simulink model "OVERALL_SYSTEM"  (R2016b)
settings: Solver=VariableStepAuto  StartTime=0.0  StopTime=12  FixedStep=0.1e-3  RelTol=1e-3
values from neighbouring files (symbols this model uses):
  beta_max = 90    [SYSTEM_PATAMETERS.m]
  beta_min = 0    [SYSTEM_PATAMETERS.m]
  beta_r = 4    [SYSTEM_PATAMETERS.m]
  c1 = 0.5    [SYSTEM_PATAMETERS.m]
  c2 = 116    [SYSTEM_PATAMETERS.m]
  c3 = 0.4    [SYSTEM_PATAMETERS.m]
  c4 = 5    [SYSTEM_PATAMETERS.m]
  c5 = 21    [SYSTEM_PATAMETERS.m]
  c6 = 0    [SYSTEM_PATAMETERS.m]
  Cdc = 0.08    [SYSTEM_PATAMETERS.m]
  Cp_max = 0.41    [SYSTEM_PATAMETERS.m]
  fn = 50    [SYSTEM_PATAMETERS.m]
  I2base = (2*Sn)/(3*V2base)    [SYSTEM_PATAMETERS.m]
  Ibase = (2*Sn)/(3*Vbase)    [SYSTEM_PATAMETERS.m]
  Idcbase = ((3/2)*Vbase*Ibase)/Vdcbase    [SYSTEM_PATAMETERS.m]
  J = Sn*2*H/(wm^2)    (= 133997.265367)    [SYSTEM_PATAMETERS.m]
  Ki = Kp/Ti    (= 750)    [SYSTEM_PATAMETERS.m]
  Ki_SSC = Kp_SSC/Ti_SSC    [SYSTEM_PATAMETERS.m]
  Kib = Kpb/Tb    (= 25)    [SYSTEM_PATAMETERS.m]
  Kibv = Kpbv/Tibv    [SYSTEM_PATAMETERS.m]
  Kidc = Kpdc/Tidc    [SYSTEM_PATAMETERS.m]
  Kiq = Kpq/Tiq    [SYSTEM_PATAMETERS.m]
  Kiw = Kpw/Tiw    (= 1)    [SYSTEM_PATAMETERS.m]
  Kp = xs_filter/(2*wbase*Ta)    (= 12.7323954474)    [SYSTEM_PATAMETERS.m]
  Kp_SSC = ls_filter/(2*wbase*Te)    [SYSTEM_PATAMETERS.m]
  Kpb = 5    [SYSTEM_PATAMETERS.m]
  Kpbv = ls_filterb/(2*wbase*Te)    [SYSTEM_PATAMETERS.m]
  Kpdc = (Vdcbase*Tc)/(V2*a*Teq)    [SYSTEM_PATAMETERS.m]
  Kpq = Tf_Q_const*rs_filter/(a*Teq)    [SYSTEM_PATAMETERS.m]
  Kpw = 4    [SYSTEM_PATAMETERS.m]
  lambda_opt = 7.95    [SYSTEM_PATAMETERS.m]
  ls = Ls/Lbase    [SYSTEM_PATAMETERS.m]
  ls_filter = Ls_filter/Lbase    [SYSTEM_PATAMETERS.m]
  Ls_filter = Xs_filter/we    [SYSTEM_PATAMETERS.m]
  polepairs = poles/2    (= 115)    [SYSTEM_PATAMETERS.m]
  psim_pu = psim/psibase    [SYSTEM_PATAMETERS.m]
  r = 26    [SYSTEM_PATAMETERS.m]
  rho = 1.225    [SYSTEM_PATAMETERS.m]
  Rs = rs*Zbase    [SYSTEM_PATAMETERS.m]
  Rs_filter = rs_filter*Zbase    [SYSTEM_PATAMETERS.m]
  Sn = 250e3    (= 250000)    [SYSTEM_PATAMETERS.m]
  Ta = Tsw/2    (= 0.0001)    [SYSTEM_PATAMETERS.m]
  Ts = 1e-5    (= 1e-05)    [SYSTEM_PATAMETERS.m]
  V2 = 400    [SYSTEM_PATAMETERS.m]
  V2base = V2*sqrt(2)/sqrt(3)    [SYSTEM_PATAMETERS.m]
  Vbase = V1*sqrt(2)/sqrt(3)    [SYSTEM_PATAMETERS.m]
  Vdcbase = 3*Vbase    [SYSTEM_PATAMETERS.m]
  w2base = 2*pi*fn    (= 314.159265359)    [SYSTEM_PATAMETERS.m]
  wbase = 2*pi*fn    (= 314.159265359)    [SYSTEM_PATAMETERS.m]
  wm = nm*pi/30    (= 2.73181969877)    [SYSTEM_PATAMETERS.m]
undefined symbols (not defined in the file or in its folder): bridge, by, dend, DiscIntNeverNeededParam, established, Flux, h, Ion, K, Ld, linkage, Lithium, Lq, magnets, numd, phase, Pm0, pulses, sigbuilder_block, Td, Three, Tlim, Tr, V
libraries: powerlib x32, powerlib_meascontrol x14, simulink x10, powerlib_extras x2, sps_avr x1, electricdrivelib x1
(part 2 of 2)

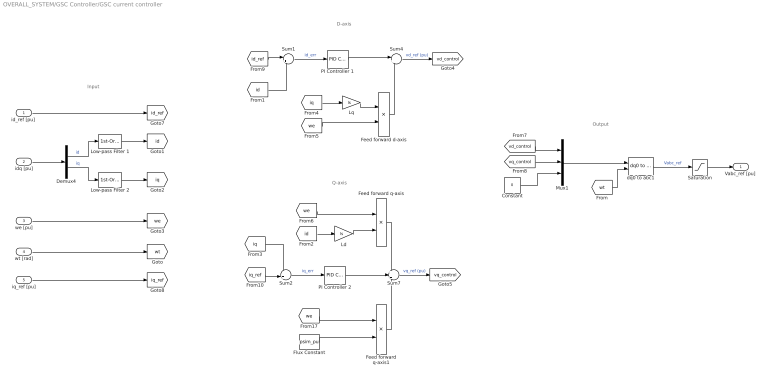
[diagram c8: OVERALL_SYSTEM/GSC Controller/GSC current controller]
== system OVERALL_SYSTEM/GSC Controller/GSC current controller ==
  note: D-axis
  note: Q-axis
  note: Input
  note: Output
  "id_ref [pu] " : Inport
  idq [pu] : Inport  Port=2
  we [pu] : Inport  Port=3
  wt [rad] : Inport  Port=4
  iq_ref [pu] : Inport  Port=5
  Constant : Constant  Value=0
  Demux4 : Demux  Outputs=2
  Feed forward d-axis : Product
  Feed forward q-axis : Product
  Feed forward q-axis1 : Product
  Flux Constant : Constant  Value=psim_pu
  Ld : Gain  Gain=ls
  Low-pass Filter 1 : powerlib_extras/Control  Blocks/1st-Order  Filter  FilterType=Lowpass  Tc=3e-4  Initialize=off  Vac_Init=[0.8 -25 50]  Vdc_Init=0  PlotResponse=off  param1=[1 2000 1]
  Low-pass Filter 2 : powerlib_extras/Control  Blocks/1st-Order  Filter  FilterType=Lowpass  Tc=3e-4  Initialize=off  Vac_Init=[0.8 -25 50]  Vdc_Init=0  PlotResponse=off  param1=[1 2000 1]
  Lq : Gain  Gain=ls
  Mux1 : Mux  Inputs=3
  PI Controller 1 : simulink/Continuous/PID Controller  Controller=PI  TimeDomain=Continuous-time  SampleTime=-1  IntegratorMethod=Forward Euler  FilterMethod=Forward Euler  Form=Parallel  UseFilter=on  ControllerParametersSource=internal  P=Kp  I=Ki  D=0  N=100  InitialConditionSource=internal  InitialConditionForIntegrator=0  InitialConditionForFilter=0  ExternalReset=none  LimitOutput=off  UpperSaturationLimit=inf  LowerSaturationLimit=-inf  LinearizeAsGain=on  AntiWindupMode=none  Kb=1  TrackingMode=off  Kt=1  PParamMin=[]  PParamMax=[]  IParamMin=[]  IParamMax=[]  DParamMin=[]  DParamMax=[]  NParamMin=[]  NParamMax=[]  KbParamMin=[]  KbParamMax=[]  KtParamMin=[]  KtParamMax=[]  POutMin=[]  POutMax=[]  IOutMin=[]  IOutMax=[]  DOutMin=[]  DOutMax=[]  NOutMin=[]  NOutMax=[]  KbOutMin=[]  KbOutMax=[]  KtOutMin=[]  KtOutMax=[]  IntegratorOutMin=[]  IntegratorOutMax=[]  FilterOutMin=[]  FilterOutMax=[]  SumOutMin=[]  SumOutMax=[]  SumI1OutMin=[]  SumI1OutMax=[]  SumI2OutMin=[]  SumI2OutMax=[]  SumI3OutMin=[]  SumI3OutMax=[]  SumDOutMin=[]  SumDOutMax=[]  SaturationOutMin=[]  SaturationOutMax=[]  IntegratorContinuousStateAttributes=''  IntegratorStateMustResolveToSignalObject=off  IntegratorRTWStateStorageClass=Auto  FilterContinuousStateAttributes=''  FilterStateMustResolveToSignalObject=off  FilterRTWStateStorageClass=Auto  DifferentiatorICPrevScaledInput=0  DifferentiatorOutMin=[]  DifferentiatorOutMax=[]
  PI Controller 2 : simulink/Continuous/PID Controller  Controller=PI  TimeDomain=Continuous-time  SampleTime=-1  IntegratorMethod=Forward Euler  FilterMethod=Forward Euler  Form=Parallel  UseFilter=on  ControllerParametersSource=internal  P=Kp  I=Ki  D=0  N=100  InitialConditionSource=internal  InitialConditionForIntegrator=0  InitialConditionForFilter=0  ExternalReset=none  LimitOutput=off  UpperSaturationLimit=inf  LowerSaturationLimit=-inf  LinearizeAsGain=on  AntiWindupMode=none  Kb=1  TrackingMode=off  Kt=1  PParamMin=[]  PParamMax=[]  IParamMin=[]  IParamMax=[]  DParamMin=[]  DParamMax=[]  NParamMin=[]  NParamMax=[]  KbParamMin=[]  KbParamMax=[]  KtParamMin=[]  KtParamMax=[]  POutMin=[]  POutMax=[]  IOutMin=[]  IOutMax=[]  DOutMin=[]  DOutMax=[]  NOutMin=[]  NOutMax=[]  KbOutMin=[]  KbOutMax=[]  KtOutMin=[]  KtOutMax=[]  IntegratorOutMin=[]  IntegratorOutMax=[]  FilterOutMin=[]  FilterOutMax=[]  SumOutMin=[]  SumOutMax=[]  SumI1OutMin=[]  SumI1OutMax=[]  SumI2OutMin=[]  SumI2OutMax=[]  SumI3OutMin=[]  SumI3OutMax=[]  SumDOutMin=[]  SumDOutMax=[]  SaturationOutMin=[]  SaturationOutMax=[]  IntegratorContinuousStateAttributes=''  IntegratorStateMustResolveToSignalObject=off  IntegratorRTWStateStorageClass=Auto  FilterContinuousStateAttributes=''  FilterStateMustResolveToSignalObject=off  FilterRTWStateStorageClass=Auto  DifferentiatorICPrevScaledInput=0  DifferentiatorOutMin=[]  DifferentiatorOutMax=[]
  Saturation : Saturate  UpperLimit=1  LowerLimit=-1
  Sum1 : Sum  Inputs=|+-
  Sum2 : Sum  Inputs=-+|
  Sum4 : Sum  Inputs=|+-
  Sum7 : Sum  Inputs=+++
  dq0 to abc1 : powerlib_meascontrol/Transformations/dq0 to abc  Alignment=Aligned with phase A axis
  "Vabc_ref [pu] " : Outport
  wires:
  PI Controller 2/1 -> Sum7/2
  Demux4/1 -> Low-pass Filter 1/1  "id"
  "id_ref [pu] "/1 -> [id_ref]
  Constant/1 -> Mux1/3
  Sum2/1 -> PI Controller 2/1  "iq_err"
  dq0 to abc1/1 -> Saturation/1  "Vabc_ref"
  Sum4/1 -> [vd_control]  "vd_ref (pu)"
  Feed forward q-axis/1 -> Sum7/1
  Mux1/1 -> dq0 to abc1/1
  Sum7/1 -> [vq_control]  "vq_ref (pu)"
  Ld/1 -> Feed forward q-axis/2
  Sum1/1 -> PI Controller 1/1  "id_err"
  Lq/1 -> Feed forward d-axis/1
  PI Controller 1/1 -> Sum4/1
  Feed forward d-axis/1 -> Sum4/2
  idq [pu]/1 -> Demux4/1
  wt [rad]/1 -> [wt]
  [wt] -> dq0 to abc1/2
  Demux4/2 -> Low-pass Filter 2/1  "iq"
  [id] -> Ld/1
  [iq] -> Lq/1
  we [pu]/1 -> [we]
  [we] -> Feed forward d-axis/2
  [we] -> Feed forward q-axis/1
  [vd_control] -> Mux1/1
  [vq_control] -> Mux1/2
  Saturation/1 -> "Vabc_ref [pu] "/1
  Flux Constant/1 -> Feed forward q-axis1/2
  [we] -> Feed forward q-axis1/1
  Feed forward q-axis1/1 -> Sum7/3
  [iq] -> Sum2/1
  [id] -> Sum1/2
  iq_ref [pu]/1 -> [iq_ref]
  Low-pass Filter 1/1 -> [id]
  Low-pass Filter 2/1 -> [iq]
  [id_ref] -> Sum1/1
  [iq_ref] -> Sum2/2

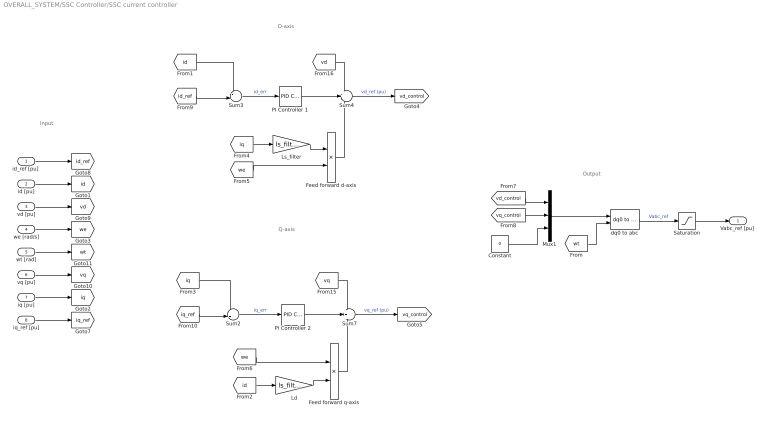
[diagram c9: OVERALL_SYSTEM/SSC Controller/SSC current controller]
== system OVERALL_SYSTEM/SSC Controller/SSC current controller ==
  note: D-axis
  note: Q-axis
  note: Input
  note: Output
  "id_ref [pu] " : Inport
  id [pu] : Inport  Port=2
  vd [pu] : Inport  Port=3
  we [rad/s] : Inport  Port=4
  wt [rad] : Inport  Port=5
  vq [pu] : Inport  Port=6
  iq [pu] : Inport  Port=7
  iq_ref [pu] : Inport  Port=8
  Constant : Constant  Value=0
  Feed forward d-axis : Product
  Feed forward q-axis : Product
  Ld : Gain  Gain=ls_filter
  Ls_filter : Gain  Gain=ls_filter
  Mux1 : Mux  Inputs=3
  PI Controller 1 : simulink/Continuous/PID Controller  Controller=PI  TimeDomain=Continuous-time  SampleTime=-1  IntegratorMethod=Forward Euler  FilterMethod=Forward Euler  Form=Parallel  UseFilter=on  ControllerParametersSource=internal  P=Kp_SSC  I=Ki_SSC  D=0.05  N=1  InitialConditionSource=internal  InitialConditionForIntegrator=0  InitialConditionForFilter=0  ExternalReset=none  LimitOutput=off  UpperSaturationLimit=inf  LowerSaturationLimit=-inf  LinearizeAsGain=on  AntiWindupMode=none  Kb=1  TrackingMode=off  Kt=1  PParamMin=[]  PParamMax=[]  IParamMin=[]  IParamMax=[]  DParamMin=[]  DParamMax=[]  NParamMin=[]  NParamMax=[]  KbParamMin=[]  KbParamMax=[]  KtParamMin=[]  KtParamMax=[]  POutMin=[]  POutMax=[]  IOutMin=[]  IOutMax=[]  DOutMin=[]  DOutMax=[]  NOutMin=[]  NOutMax=[]  KbOutMin=[]  KbOutMax=[]  KtOutMin=[]  KtOutMax=[]  IntegratorOutMin=[]  IntegratorOutMax=[]  FilterOutMin=[]  FilterOutMax=[]  SumOutMin=[]  SumOutMax=[]  SumI1OutMin=[]  SumI1OutMax=[]  SumI2OutMin=[]  SumI2OutMax=[]  SumI3OutMin=[]  SumI3OutMax=[]  SumDOutMin=[]  SumDOutMax=[]  SaturationOutMin=[]  SaturationOutMax=[]  IntegratorContinuousStateAttributes=''  IntegratorStateMustResolveToSignalObject=off  IntegratorRTWStateStorageClass=Auto  FilterContinuousStateAttributes=''  FilterStateMustResolveToSignalObject=off  FilterRTWStateStorageClass=Auto  DifferentiatorICPrevScaledInput=0  DifferentiatorOutMin=[]  DifferentiatorOutMax=[]
  PI Controller 2 : simulink/Continuous/PID Controller  Controller=PI  TimeDomain=Continuous-time  SampleTime=-1  IntegratorMethod=Forward Euler  FilterMethod=Forward Euler  Form=Parallel  UseFilter=on  ControllerParametersSource=internal  P=Kp_SSC  I=Ki_SSC  D=0  N=100  InitialConditionSource=internal  InitialConditionForIntegrator=0  InitialConditionForFilter=0  ExternalReset=none  LimitOutput=off  UpperSaturationLimit=inf  LowerSaturationLimit=-inf  LinearizeAsGain=on  AntiWindupMode=none  Kb=1  TrackingMode=off  Kt=1  PParamMin=[]  PParamMax=[]  IParamMin=[]  IParamMax=[]  DParamMin=[]  DParamMax=[]  NParamMin=[]  NParamMax=[]  KbParamMin=[]  KbParamMax=[]  KtParamMin=[]  KtParamMax=[]  POutMin=[]  POutMax=[]  IOutMin=[]  IOutMax=[]  DOutMin=[]  DOutMax=[]  NOutMin=[]  NOutMax=[]  KbOutMin=[]  KbOutMax=[]  KtOutMin=[]  KtOutMax=[]  IntegratorOutMin=[]  IntegratorOutMax=[]  FilterOutMin=[]  FilterOutMax=[]  SumOutMin=[]  SumOutMax=[]  SumI1OutMin=[]  SumI1OutMax=[]  SumI2OutMin=[]  SumI2OutMax=[]  SumI3OutMin=[]  SumI3OutMax=[]  SumDOutMin=[]  SumDOutMax=[]  SaturationOutMin=[]  SaturationOutMax=[]  IntegratorContinuousStateAttributes=''  IntegratorStateMustResolveToSignalObject=off  IntegratorRTWStateStorageClass=Auto  FilterContinuousStateAttributes=''  FilterStateMustResolveToSignalObject=off  FilterRTWStateStorageClass=Auto  DifferentiatorICPrevScaledInput=0  DifferentiatorOutMin=[]  DifferentiatorOutMax=[]
  Saturation : Saturate  UpperLimit=1  LowerLimit=-1
  Sum2 : Sum  Inputs=-+|
  Sum3 : Sum  Inputs=-+|
  Sum4 : Sum  Inputs=++-
  Sum7 : Sum  Inputs=+++
  dq0 to abc : powerlib_meascontrol/Transformations/dq0 to abc  Alignment=90 degrees behind phase A axis
  "Vabc_ref [pu] " : Outport
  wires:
  PI Controller 2/1 -> Sum7/2
  "id_ref [pu] "/1 -> [id_ref]
  Constant/1 -> Mux1/3
  Sum2/1 -> PI Controller 2/1  "iq_err"
  dq0 to abc/1 -> Saturation/1  "Vabc_ref"
  Sum4/1 -> [vd_control]  "vd_ref (pu)"
  Mux1/1 -> dq0 to abc/1
  Sum7/1 -> [vq_control]  "vq_ref (pu)"
  Sum3/1 -> PI Controller 1/1  "id_err"
  iq_ref [pu]/1 -> [iq_ref]
  Ls_filter/1 -> Feed forward d-axis/1
  [wt] -> dq0 to abc/2
  [iq] -> Sum2/1
  [iq] -> Ls_filter/1
  [we] -> Feed forward d-axis/2
  [vd_control] -> Mux1/1
  [vq_control] -> Mux1/2
  Saturation/1 -> "Vabc_ref [pu] "/1
  Feed forward d-axis/1 -> Sum4/3
  PI Controller 1/1 -> Sum4/2
  [vd] -> Sum4/1
  id [pu]/1 -> [id]
  iq [pu]/1 -> [iq]
  wt [rad]/1 -> [wt]
  vd [pu]/1 -> [vd]
  vq [pu]/1 -> [vq]
  we [rad/s]/1 -> [we]
  [id] -> Sum3/1
  [vq] -> Sum7/1
  [id_ref] -> Sum3/2
  [iq_ref] -> Sum2/2
  Feed forward q-axis/1 -> Sum7/3
  Ld/1 -> Feed forward q-axis/2
  [id] -> Ld/1
  [we] -> Feed forward q-axis/1

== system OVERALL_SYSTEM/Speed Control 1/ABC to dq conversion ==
  Iabc : Inport
  Teta : Inport  Port=2
  Fcn : Fcn  Expr=sin(u)
  Fcn1 : Fcn  Expr=cos(u)
  Gain : Gain  Gain=2/3
  Gain1 : Gain  Gain=2/3
  Mux : Mux  Inputs=[1 1 3]
  id : Fcn  Expr=u[1]*u[3]+(1.7320508*u[2]-u[1])*u[4]*0.5+(-u[1]-1.7320508*u[2])*u[5]*0.5
  iq : Fcn  Expr=-u[2]*u[3]+(u[2]+1.7320508*u[1])*u[4]*0.5+(u[2]-1.7320508*u[1])*u[5]*0.5
  Id : Outport  InitialOutput=0
  Iq : Outport  Port=2  InitialOutput=0
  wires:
  Fcn/1 -> Mux/2
  Fcn1/1 -> Mux/1
  Teta/1 -> Fcn1/1, Fcn/1
  Mux/1 -> iq/1, id/1
  Iabc/1 -> Mux/3
  iq/1 -> Gain1/1
  id/1 -> Gain/1
  Gain/1 -> Id/1
  Gain1/1 -> Iq/1

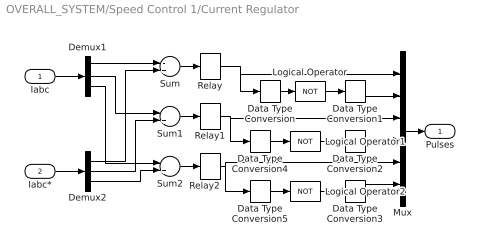
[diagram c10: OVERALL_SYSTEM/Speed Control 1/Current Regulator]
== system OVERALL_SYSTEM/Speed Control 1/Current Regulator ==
  Iabc : Inport
  Iabc* : Inport  Port=2
  Data Type Conversion : DataTypeConversion  OutDataTypeStr=boolean
  Data Type Conversion1 : DataTypeConversion  OutDataTypeStr=double
  Data Type Conversion2 : DataTypeConversion  OutDataTypeStr=double
  Data Type Conversion3 : DataTypeConversion  OutDataTypeStr=double
  Data Type Conversion4 : DataTypeConversion  OutDataTypeStr=boolean
  Data Type Conversion5 : DataTypeConversion  OutDataTypeStr=boolean
  Demux1 : Demux  Outputs=3
  Demux2 : Demux  Outputs=3
  Logical Operator : Logic  Operator=NOT
  Logical Operator1 : Logic  Operator=NOT
  Logical Operator2 : Logic  Operator=NOT
  Mux : Mux  Inputs=6
  Relay : Relay  OnSwitchValue=h/2  OffSwitchValue=-h/2
  Relay1 : Relay  OnSwitchValue=h/2  OffSwitchValue=-h/2
  Relay2 : Relay  OnSwitchValue=h/2  OffSwitchValue=-h/2
  Sum : Sum  Inputs=-+
  Sum1 : Sum  Inputs=-+
  Sum2 : Sum  Inputs=-+
  Pulses : Outport  InitialOutput=0
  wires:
  Sum/1 -> Relay/1
  Sum1/1 -> Relay1/1
  Demux1/1 -> Sum/1
  Demux1/2 -> Sum1/1
  Mux/1 -> Pulses/1
  Iabc/1 -> Demux1/1
  Sum2/1 -> Relay2/1
  Demux1/3 -> Sum2/1
  Demux2/3 -> Sum2/2
  Demux2/2 -> Sum1/2
  Demux2/1 -> Sum/2
  Iabc*/1 -> Demux2/1
  Relay/1 -> Mux/1, Data Type Conversion/1
  Relay1/1 -> Mux/3, Data Type Conversion4/1
  Relay2/1 -> Mux/5, Data Type Conversion5/1
  Data Type Conversion/1 -> Logical Operator/1
  Logical Operator/1 -> Data Type Conversion1/1
  Data Type Conversion1/1 -> Mux/2
  Logical Operator1/1 -> Data Type Conversion2/1
  Data Type Conversion2/1 -> Mux/4
  Logical Operator2/1 -> Data Type Conversion3/1
  Data Type Conversion3/1 -> Mux/6
  Data Type Conversion4/1 -> Logical Operator1/1
  Data Type Conversion5/1 -> Logical Operator2/1

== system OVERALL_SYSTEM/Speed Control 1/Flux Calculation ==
  note: Phir = Lm *Id / (1 +Tr .s)
  note: Lm = 34.7 mH
  note: Lr = Ll'r +Lm = 0.8 +34.7= 35.5 mH
  note: Tr = Lr / Rr = 0.1557 s
  note: Rr = 0.228 ohms
  Id : Inport
  Discrete Tranfer Function : Subsystem
  Lm : Gain  Gain=34.7e-3
  Phir : Outport
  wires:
  Discrete Tranfer Function/1(Out) -> Phir/1
  Id/1 -> Lm/1
  Lm/1 -> Discrete Tranfer Function/1(In)

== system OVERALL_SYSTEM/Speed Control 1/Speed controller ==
  w : Inport
  w* : Inport  Port=2
  Discrete-Time Integrator : DiscreteIntegrator  IntegratorMethod=Integration: Trapezoidal  SampleTime=Ts  LimitOutput=on  UpperSaturationLimit=Tlim  LowerSaturationLimit=-Tlim  ICPrevOutput=DiscIntNeverNeededParam  ICPrevScaledInput=DiscIntNeverNeededParam
  Gain : Gain  Gain=Ki
  Gain1 : Gain  Gain=Kp
  Saturation : Saturate  UpperLimit=Tlim  LowerLimit=-Tlim
  Sum1 : Sum  Inputs=+-
  Sum2 : Sum
  Te* : Outport  InitialOutput=0
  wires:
  Gain1/1 -> Sum2/1
  Gain/1 -> Discrete-Time Integrator/1
  Sum1/1 -> Gain/1, Gain1/1
  Discrete-Time Integrator/1 -> Sum2/2
  Sum2/1 -> Saturation/1
  Saturation/1 -> Te*/1
  w/1 -> Sum1/2
  w*/1 -> Sum1/1

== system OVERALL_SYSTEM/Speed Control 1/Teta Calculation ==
  note: Teta= Electrical angle= integ ( wr + wm)
  note: wr = Rotor frequency (rad/s) = Lm *Iq / ( Tr * Phir)
  note: Lm = 34.7 mH
  note: Rr= 0.228 ohms
  note: Lr = Ll'r +Lm = 0.8 +34.7= 35.5 mH
  note: wm= Rotor mechanical speed (rad/s)
  note: Tr = Lr / Rr = 0.1557 s
  Phir : Inport
  wm : Inport  Port=2
  Iq : Inport  Port=3
  Discrete-Time Integrator : DiscreteIntegrator  SampleTime=Ts  ICPrevOutput=DiscIntNeverNeededParam  ICPrevScaledInput=DiscIntNeverNeededParam
  Fcn : Fcn  Expr=34.7e-3*u[1]/(u[2]*0.1557+1e-3)
  Gain2 : Gain
  Gain3 : Gain  Gain=2
  Mux : Mux  Inputs=2
  Sum : Sum
  Teta : Outport  InitialOutput=0
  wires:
  Discrete-Time Integrator/1 -> Teta/1
  Sum/1 -> Discrete-Time Integrator/1
  Gain3/1 -> Sum/2
  Gain2/1 -> Sum/1
  wm/1 -> Gain3/1
  Fcn/1 -> Gain2/1
  Phir/1 -> Mux/2
  Iq/1 -> Mux/1
  Mux/1 -> Fcn/1

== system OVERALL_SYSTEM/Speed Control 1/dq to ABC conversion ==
  Teta : Inport
  Id* : Inport  Port=2
  Iq* : Inport  Port=3
  Fcn : Fcn  Expr=sin(u)
  Fcn1 : Fcn  Expr=cos(u)
  Gain2 : Gain
  Gain3 : Gain
  Gain4 : Gain
  Mux : Mux
  Mux2 : Mux  Inputs=3
  ia : Fcn  Expr=-u[3]*u[2] + u[4]*u[1]
  ib : Fcn  Expr=(-u[1]+1.7320508*u[2])*u[4]*0.5+(u[2]+1.7320508*u[1])*u[3]*0.5
  ic : Sum  Inputs=--
  Iabc* : Outport  InitialOutput=0
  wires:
  Fcn/1 -> Mux/2
  Fcn1/1 -> Mux/1
  Mux2/1 -> Iabc*/1
  Mux/1 -> ib/1, ia/1
  Teta/1 -> Fcn1/1, Fcn/1
  Iq*/1 -> Mux/3
  Id*/1 -> Mux/4
  Gain3/1 -> Mux2/2
  ic/1 -> Gain4/1
  Gain4/1 -> Mux2/3
  Gain2/1 -> Mux2/1
  ia/1 -> Gain2/1, ic/2
  ib/1 -> Gain3/1, ic/1

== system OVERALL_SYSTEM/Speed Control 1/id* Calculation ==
  note: Id* = Phir*/ Lm
  note: Lm= 34.7 mH
  Phir* : Inport
  KF : Gain  Gain=1/34.7e-3
  Id* : Outport
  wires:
  KF/1 -> Id*/1
  Phir*/1 -> KF/1

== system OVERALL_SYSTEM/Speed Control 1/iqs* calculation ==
  note: Iq= ( 2/3) * (2/p) * ( Lr/Lm) * (Te / Phir)
  note: Lm = 34.7 mH
  note: Lr = Ll'r +Lm = 0.8 +34.7= 35.5 mH
  note: p= nb of poles = 4
  note: Iq= 0.341 * (Te / Phir)
  Phir : Inport
  Te* : Inport  Port=2
  Fcn : Fcn  Expr=u[1]*0.341/(u[2]+1e-3)
  Mux1 : Mux  Inputs=2
  Iq* : Outport  InitialOutput=0
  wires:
  Phir/1 -> Mux1/2
  Fcn/1 -> Iq*/1
  Te*/1 -> Mux1/1
  Mux1/1 -> Fcn/1

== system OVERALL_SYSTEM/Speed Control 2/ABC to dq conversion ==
  Iabc : Inport
  Teta : Inport  Port=2
  Fcn : Fcn  Expr=sin(u)
  Fcn1 : Fcn  Expr=cos(u)
  Gain : Gain  Gain=2/3
  Gain1 : Gain  Gain=2/3
  Mux : Mux  Inputs=[1 1 3]
  id : Fcn  Expr=u[1]*u[3]+(1.7320508*u[2]-u[1])*u[4]*0.5+(-u[1]-1.7320508*u[2])*u[5]*0.5
  iq : Fcn  Expr=-u[2]*u[3]+(u[2]+1.7320508*u[1])*u[4]*0.5+(u[2]-1.7320508*u[1])*u[5]*0.5
  Id : Outport  InitialOutput=0
  Iq : Outport  Port=2  InitialOutput=0
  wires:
  Fcn/1 -> Mux/2
  Fcn1/1 -> Mux/1
  Teta/1 -> Fcn1/1, Fcn/1
  Mux/1 -> iq/1, id/1
  Iabc/1 -> Mux/3
  iq/1 -> Gain1/1
  id/1 -> Gain/1
  Gain/1 -> Id/1
  Gain1/1 -> Iq/1

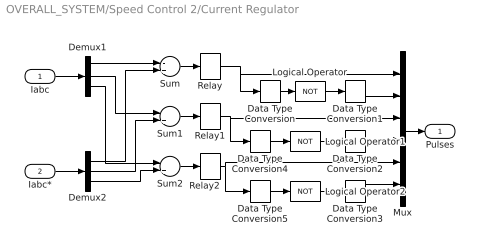
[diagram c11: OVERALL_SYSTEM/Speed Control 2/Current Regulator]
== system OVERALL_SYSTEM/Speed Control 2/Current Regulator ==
  Iabc : Inport
  Iabc* : Inport  Port=2
  Data Type Conversion : DataTypeConversion  OutDataTypeStr=boolean
  Data Type Conversion1 : DataTypeConversion  OutDataTypeStr=double
  Data Type Conversion2 : DataTypeConversion  OutDataTypeStr=double
  Data Type Conversion3 : DataTypeConversion  OutDataTypeStr=double
  Data Type Conversion4 : DataTypeConversion  OutDataTypeStr=boolean
  Data Type Conversion5 : DataTypeConversion  OutDataTypeStr=boolean
  Demux1 : Demux  Outputs=3
  Demux2 : Demux  Outputs=3
  Logical Operator : Logic  Operator=NOT
  Logical Operator1 : Logic  Operator=NOT
  Logical Operator2 : Logic  Operator=NOT
  Mux : Mux  Inputs=6
  Relay : Relay  OnSwitchValue=h/2  OffSwitchValue=-h/2
  Relay1 : Relay  OnSwitchValue=h/2  OffSwitchValue=-h/2
  Relay2 : Relay  OnSwitchValue=h/2  OffSwitchValue=-h/2
  Sum : Sum  Inputs=-+
  Sum1 : Sum  Inputs=-+
  Sum2 : Sum  Inputs=-+
  Pulses : Outport  InitialOutput=0
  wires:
  Sum/1 -> Relay/1
  Sum1/1 -> Relay1/1
  Demux1/1 -> Sum/1
  Demux1/2 -> Sum1/1
  Mux/1 -> Pulses/1
  Iabc/1 -> Demux1/1
  Sum2/1 -> Relay2/1
  Demux1/3 -> Sum2/1
  Demux2/3 -> Sum2/2
  Demux2/2 -> Sum1/2
  Demux2/1 -> Sum/2
  Iabc*/1 -> Demux2/1
  Relay/1 -> Mux/1, Data Type Conversion/1
  Relay1/1 -> Mux/3, Data Type Conversion4/1
  Relay2/1 -> Mux/5, Data Type Conversion5/1
  Data Type Conversion/1 -> Logical Operator/1
  Logical Operator/1 -> Data Type Conversion1/1
  Data Type Conversion1/1 -> Mux/2
  Logical Operator1/1 -> Data Type Conversion2/1
  Data Type Conversion2/1 -> Mux/4
  Logical Operator2/1 -> Data Type Conversion3/1
  Data Type Conversion3/1 -> Mux/6
  Data Type Conversion4/1 -> Logical Operator1/1
  Data Type Conversion5/1 -> Logical Operator2/1

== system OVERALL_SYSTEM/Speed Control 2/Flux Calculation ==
  note: Phir = Lm *Id / (1 +Tr .s)
  note: Lm = 34.7 mH
  note: Lr = Ll'r +Lm = 0.8 +34.7= 35.5 mH
  note: Tr = Lr / Rr = 0.1557 s
  note: Rr = 0.228 ohms
  Id : Inport
  Discrete Tranfer Function : Subsystem
  Lm : Gain  Gain=34.7e-3
  Phir : Outport
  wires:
  Discrete Tranfer Function/1(Out) -> Phir/1
  Id/1 -> Lm/1
  Lm/1 -> Discrete Tranfer Function/1(In)

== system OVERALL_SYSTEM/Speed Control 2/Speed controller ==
  w : Inport
  w* : Inport  Port=2
  Discrete-Time Integrator : DiscreteIntegrator  IntegratorMethod=Integration: Trapezoidal  SampleTime=Ts  LimitOutput=on  UpperSaturationLimit=Tlim  LowerSaturationLimit=-Tlim  ICPrevOutput=DiscIntNeverNeededParam  ICPrevScaledInput=DiscIntNeverNeededParam
  Gain : Gain  Gain=Ki
  Gain1 : Gain  Gain=Kp
  Saturation : Saturate  UpperLimit=Tlim  LowerLimit=-Tlim
  Sum1 : Sum  Inputs=+-
  Sum2 : Sum
  Te* : Outport  InitialOutput=0
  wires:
  Gain1/1 -> Sum2/1
  Gain/1 -> Discrete-Time Integrator/1
  Sum1/1 -> Gain/1, Gain1/1
  Discrete-Time Integrator/1 -> Sum2/2
  Sum2/1 -> Saturation/1
  Saturation/1 -> Te*/1
  w/1 -> Sum1/2
  w*/1 -> Sum1/1

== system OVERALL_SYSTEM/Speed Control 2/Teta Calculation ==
  note: Teta= Electrical angle= integ ( wr + wm)
  note: wr = Rotor frequency (rad/s) = Lm *Iq / ( Tr * Phir)
  note: Lm = 34.7 mH
  note: Rr= 0.228 ohms
  note: Lr = Ll'r +Lm = 0.8 +34.7= 35.5 mH
  note: wm= Rotor mechanical speed (rad/s)
  note: Tr = Lr / Rr = 0.1557 s
  Phir : Inport
  wm : Inport  Port=2
  Iq : Inport  Port=3
  Discrete-Time Integrator : DiscreteIntegrator  SampleTime=Ts  ICPrevOutput=DiscIntNeverNeededParam  ICPrevScaledInput=DiscIntNeverNeededParam
  Fcn : Fcn  Expr=34.7e-3*u[1]/(u[2]*0.1557+1e-3)
  Gain2 : Gain
  Gain3 : Gain  Gain=2
  Mux : Mux  Inputs=2
  Sum : Sum
  Teta : Outport  InitialOutput=0
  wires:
  Discrete-Time Integrator/1 -> Teta/1
  Sum/1 -> Discrete-Time Integrator/1
  Gain3/1 -> Sum/2
  Gain2/1 -> Sum/1
  wm/1 -> Gain3/1
  Fcn/1 -> Gain2/1
  Phir/1 -> Mux/2
  Iq/1 -> Mux/1
  Mux/1 -> Fcn/1

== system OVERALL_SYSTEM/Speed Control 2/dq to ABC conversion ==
  Teta : Inport
  Id* : Inport  Port=2
  Iq* : Inport  Port=3
  Fcn : Fcn  Expr=sin(u)
  Fcn1 : Fcn  Expr=cos(u)
  Gain2 : Gain
  Gain3 : Gain
  Gain4 : Gain
  Mux : Mux
  Mux2 : Mux  Inputs=3
  ia : Fcn  Expr=-u[3]*u[2] + u[4]*u[1]
  ib : Fcn  Expr=(-u[1]+1.7320508*u[2])*u[4]*0.5+(u[2]+1.7320508*u[1])*u[3]*0.5
  ic : Sum  Inputs=--
  Iabc* : Outport  InitialOutput=0
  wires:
  Fcn/1 -> Mux/2
  Fcn1/1 -> Mux/1
  Mux2/1 -> Iabc*/1
  Mux/1 -> ib/1, ia/1
  Teta/1 -> Fcn1/1, Fcn/1
  Iq*/1 -> Mux/3
  Id*/1 -> Mux/4
  Gain3/1 -> Mux2/2
  ic/1 -> Gain4/1
  Gain4/1 -> Mux2/3
  Gain2/1 -> Mux2/1
  ia/1 -> Gain2/1, ic/2
  ib/1 -> Gain3/1, ic/1

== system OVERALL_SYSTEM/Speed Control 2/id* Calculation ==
  note: Id* = Phir*/ Lm
  note: Lm= 34.7 mH
  Phir* : Inport
  KF : Gain  Gain=1/34.7e-3
  Id* : Outport
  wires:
  KF/1 -> Id*/1
  Phir*/1 -> KF/1

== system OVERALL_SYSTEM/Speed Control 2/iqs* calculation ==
  note: Iq= ( 2/3) * (2/p) * ( Lr/Lm) * (Te / Phir)
  note: Lm = 34.7 mH
  note: Lr = Ll'r +Lm = 0.8 +34.7= 35.5 mH
  note: p= nb of poles = 4
  note: Iq= 0.341 * (Te / Phir)
  Phir : Inport
  Te* : Inport  Port=2
  Fcn : Fcn  Expr=u[1]*0.341/(u[2]+1e-3)
  Mux1 : Mux  Inputs=2
  Iq* : Outport  InitialOutput=0
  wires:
  Phir/1 -> Mux1/2
  Fcn/1 -> Iq*/1
  Te*/1 -> Mux1/1
  Mux1/1 -> Fcn/1

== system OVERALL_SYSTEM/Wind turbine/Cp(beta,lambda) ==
  lambda : Inport
  beta : Inport  Port=2
  Mux : Mux  Inputs=2
  Mux1 : Mux  Inputs=3
  cp : Fcn  Expr=c1*(c2/u[2]-c3*u[3]-c4)*exp(-c5/u[2])+c6*u[1]
  lambda_opt : Fcn  Expr=1/(1/(u[1]+0.08*u[2])-0.035/(u[2]^3+1))
  Cp : Outport
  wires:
  lambda_opt/1 -> Mux1/2  "lambda_i"
  cp/1 -> Cp/1
  lambda/1 -> Mux1/1, Mux/1
  Mux1/1 -> cp/1
  beta/1 -> Mux1/3, Mux/2
  Mux/1 -> lambda_opt/1

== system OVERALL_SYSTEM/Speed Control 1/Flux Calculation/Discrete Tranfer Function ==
  In : Inport
  Discrete Transfer Fcn : DiscreteTransferFcn  Numerator=numd  Denominator=dend  SampleTime=Ts
  Out : Outport  InitialOutput=0
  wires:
  Discrete Transfer Fcn/1 -> Out/1
  In/1 -> Discrete Transfer Fcn/1

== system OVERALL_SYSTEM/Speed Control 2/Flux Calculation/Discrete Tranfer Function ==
  In : Inport
  Discrete Transfer Fcn : DiscreteTransferFcn  Numerator=numd  Denominator=dend  SampleTime=Ts
  Out : Outport  InitialOutput=0
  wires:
  Discrete Transfer Fcn/1 -> Out/1
  In/1 -> Discrete Transfer Fcn/1
